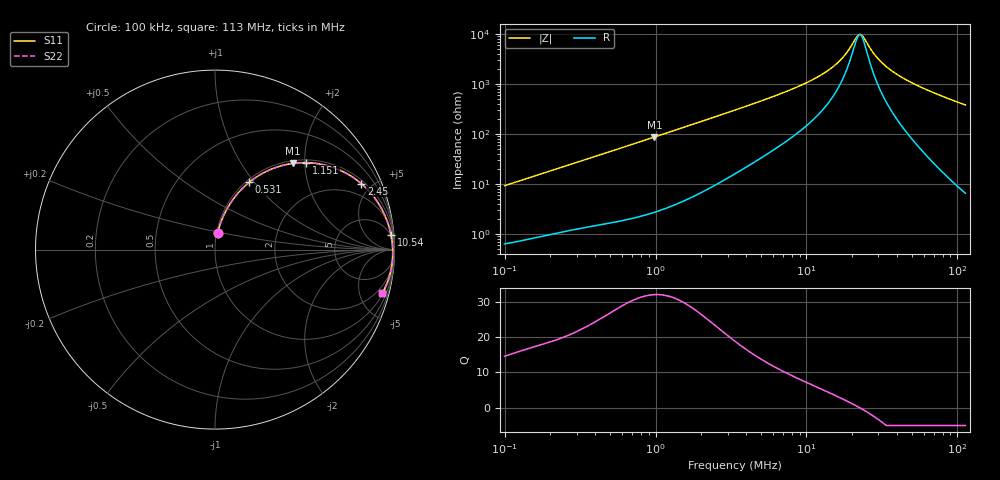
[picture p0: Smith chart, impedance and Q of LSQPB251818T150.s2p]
! LSQPB251818T150  S-PARAMETER MODEL  ( General Type )
! Model Generated by TAIYO YUDEN Corporation (http://www.ty-top.com)
! Version 2.0
! TAIYO YUDEN Control No. 100810NG19SB-FKC
! Copyright(c) 2009 TAIYO YUDEN CO.,LTD. All Rights Reserved.
! Product Description (link to TY-COMPAS)
! https://ds.yuden.co.jp/TYCOMPAS/or/detail?pn=LSQPB251818T150K&u=M
! Products Name : Inductors
! Characteristics :
!  Inductance : 15 uH , SRF(min) : 13 MHz , DC Resistance(max) : 0.559 Ohm
!  Rated Current : Saturation :760 mA , Temp Rise : 550 mA (40 degC)
!  Case Size : 2.5 x 1.8 / 0.098 x 0.071 [mm/inch] , Thickness : 1.8 / 0.071 [mm/inch]
!  (Conditions: Temperature = 25 degC , DC Bias Current/Voltage = 0A / 0V)
! External Node Assignments :
!  1  o---GGG---o  2
! GND o---------o GND
! Frequency Range : 0.1MHz  -  113.020708MHz  [ 402 STEP ]
# MHz S RI R 50
! Freq[MHz].  S11 Real  S11 Imag  S21 Real  S21 Imag  S12 Real  S12 Imag  S22 Real  S22 Imag
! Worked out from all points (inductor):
!   401 points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, 100 kHz to 113 MHz, reference 50 ohm
!   read as one part in series: L = 14.6 uH near 103.6 kHz
!   highest Q = 32.1 at 982.4 kHz (marker M1), where L = 14.1 uH
!   self-resonance near 22.44 MHz
!   S11 on the Smith chart (normalised r, x): 100 kHz: 1.01, +0.18; 531 kHz: 1.03, +0.94; 1.151 MHz: 1.06, +2.03; 2.45 MHz: 1.18, +4.35; 10.54 MHz: 4, +23; 113 MHz: 1.13, -7.61
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0.1  0.0145 0.0902  0.9855 -0.0902  0.9855 -0.0902  0.0145 0.0902
0.324641  0.088 0.2618  0.912 -0.2618  0.912 -0.2618  0.088 0.2618
0.531037  0.1907 0.3752  0.8093 -0.3752  0.8093 -0.3752  0.1907 0.3752
0.982373  0.4322 0.48  0.5678 -0.48  0.5678 -0.48  0.4322 0.48
1.053921  0.4658 0.4835  0.5342 -0.4835  0.5342 -0.4835  0.4658 0.4835
1.150727  0.5083 0.4845  0.4917 -0.4845  0.4917 -0.4845  0.5083 0.4845
1.606932  0.6637 0.4557  0.3363 -0.4557  0.3363 -0.4557  0.6637 0.4557
2.450117  0.8155 0.3672  0.1845 -0.3672  0.1845 -0.3672  0.8155 0.3672
3.421463  0.8912 0.2856  0.1088 -0.2856  0.1088 -0.2856  0.8912 0.2856
6.55585  0.9613 0.1526  0.0387 -0.1526  0.0387 -0.1526  0.9613 0.1526
10.53701  0.9802 0.0837  0.0198 -0.0837  0.0198 -0.0837  0.9802 0.0837
10.91398  0.9811 0.0793  0.0189 -0.0793  0.0189 -0.0793  0.9811 0.0793
13.71547  0.9855 0.0525  0.0145 -0.0525  0.0145 -0.0525  0.9855 0.0525
16.35082  0.9878 0.0334  0.0122 -0.0334  0.0122 -0.0334  0.9878 0.0334
18.4914  0.9889 0.0205  0.0111 -0.0205  0.0111 -0.0205  0.9889 0.0205
21.66037  0.9898 0.00419  0.0102 -0.00419  0.0102 -0.00419  0.9898 0.00419
22.43529  0.9899 0.00058  0.0101 -0.00058  0.0101 -0.00058  0.9899 0.00058
23.64996  0.9901 -0.00485  0.00995 0.00485  0.00995 0.00485  0.9901 -0.00485
29.72063  0.99 -0.0289  0.00997 0.0289  0.00997 0.0289  0.99 -0.0289
35.43129  0.9892 -0.0486  0.0108 0.0486  0.0108 0.0486  0.9892 -0.0486
55.95543  0.9813 -0.1088  0.0187 0.1088  0.0187 0.1088  0.9813 -0.1088
113.0207  0.9318 -0.2437  0.0682 0.2437  0.0682 0.2437  0.9318 -0.2437
